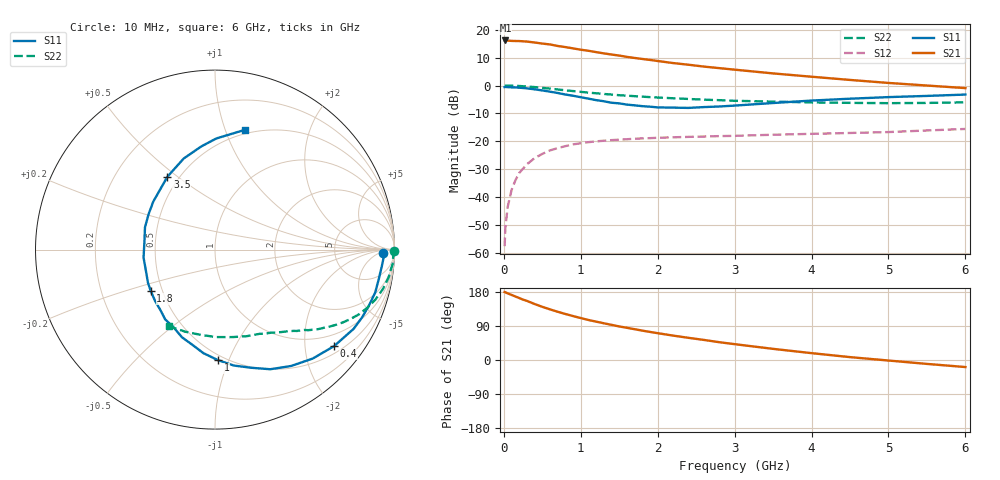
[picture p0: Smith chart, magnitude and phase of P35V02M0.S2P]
! SIEMENS Small Signal Semiconductors
! BFP181
! Si NPN RF Bipolar Junction Transistor in SOT143
! VCE = 5 V  IC = 2 mA
! Common Emitter S-Parameters:  March  1996
# GHz  S  MA  R  50
!  f  S11  S21  S12  S22
! GHz  MAG  ANG  MAG  ANG  MAG  ANG  MAG  ANG
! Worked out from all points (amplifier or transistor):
!   36 points, 10 MHz to 6 GHz, reference 50 ohm
!   highest |S21| = 16.2 dB at 20 MHz (marker M1)
!   |S21| within 3 dB of that: start of sweep to 932 MHz
!   unconditionally stable (mu >= 1): 2.514 GHz to end of sweep
!   at 250 MHz: K = 0.13, MSG = 22.9 dB, |S12| = -29.8 dB
!   at 1.4 GHz: K = 0.63, MSG = 15.4 dB, |S12| = -19.6 dB
!   at 6 GHz: K = 1.13, MAG = 5.2 dB, |S12| = -15.6 dB
!   lowest NFmin = 1.35 dB at 450 MHz
!   S11 on the Smith chart (normalised r, x): 10 MHz: 29, -8; 400 MHz: 0.67, -2.67; 1 GHz: 0.46, -0.91; 1.8 GHz: 0.43, -0.24; 3.5 GHz: 0.43, +0.46; 6 GHz: 0.46, +1.17
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0.01  0.9372 -1.0  6.433 179.3  0.0013 82.0  0.9969 -0.3
0.02  0.9415 -2.2  6.445 178.8  0.0028 81.3  0.9903 -0.9
0.05  0.9356 -5.0  6.399 175.8  0.0066 90.8  0.9936 -2.3
0.1  0.9272 -10.1  6.33 171.8  0.0132 80.2  0.9931 -4.6
0.15  0.9241 -15.0  6.302 167.6  0.0198 79.9  0.9849 -6.8
0.25  0.9025 -24.7  6.223 159.3  0.0322 74.7  0.9695 -11.2
0.3  0.8894 -29.8  6.151 156.0  0.0385 71.9  0.9604 -13.3
0.4  0.8541 -39.0  5.925 147.7  0.0496 66.8  0.9364 -17.3
0.5  0.8155 -48.1  5.665 140.3  0.0591 61.0  0.9085 -20.9
0.6  0.7749 -56.8  5.462 133.6  0.0683 56.7  0.8785 -24.3
0.8  0.6889 -72.9  4.899 121.4  0.0814 48.8  0.8206 -29.6
1  0.616 -88.5  4.397 110.7  0.0918 42.4  0.7691 -33.9
1.1  0.5805 -96.4  4.206 105.6  0.096 39.9  0.7455 -35.8
1.3  0.5217 -110.7  3.777 96.9  0.1019 34.9  0.7048 -39.3
1.5  0.4774 -125.6  3.45 88.5  0.1062 31.7  0.6692 -42.0
1.8  0.4256 -147.3  2.999 77.5  0.1122 27.7  0.6305 -45.9
2.2  0.4005 -173.7  2.531 64.4  0.1174 23.4  0.5901 -51.1
2.8  0.4196 151.7  2.052 47.0  0.1233 19.4  0.5455 -59.2
3.5  0.4847 123.2  1.649 29.4  0.1305 16.4  0.514 -69.8
4.5  0.5793 97.7  1.259 7.6  0.1404 12.8  0.4876 -89.0
5.5  0.6501 82.1  0.999 -10.3  0.1558 11.5  0.4865 -110.0
6  0.6876 76.0  0.898 -18.6  0.1658 9.5  0.4979 -120.9
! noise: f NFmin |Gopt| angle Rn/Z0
0.45  1.35  0.6  17  0.4
0.9  1.45  0.5  36  0.4
1.8  1.8  0.31  80  0.37
